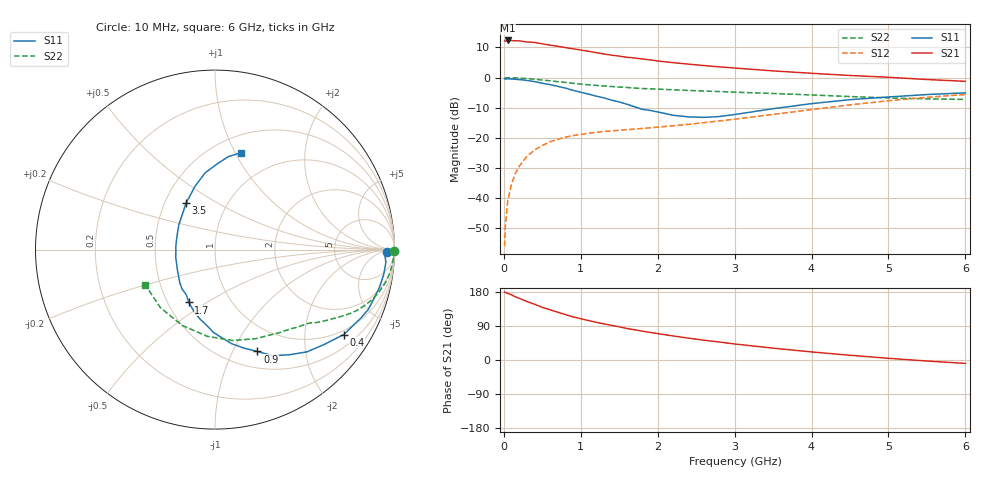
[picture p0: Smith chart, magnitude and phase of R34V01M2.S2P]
! SIEMENS Small Signal Semiconductors
! BFR181
! Si NPN RF Bipolar Junction Transistor in SOT23
! VCE = 4 V  IC = 1.2 mA
! Common Emitter S-Parameters:  May  1996
# GHz  S  MA  R  50
!  f  S11  S21  S12  S22
! GHz  MAG  ANG  MAG  ANG  MAG  ANG  MAG  ANG
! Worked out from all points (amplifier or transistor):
!   36 points, 10 MHz to 6 GHz, reference 50 ohm
!   highest |S21| = 12.3 dB at 50 MHz (marker M1)
!   |S21| within 3 dB of that: start of sweep to 957.6 MHz
!   unconditionally stable (mu >= 1): 1.924 GHz to 3.596 GHz
!   at 250 MHz: K = 0.17, MSG = 19.8 dB, |S12| = -27.7 dB
!   at 1.4 GHz: K = 0.82, MSG = 12.6 dB, |S12| = -17.7 dB
!   at 6 GHz: K = 0.87, MSG = 2.2 dB, |S12| = -5.6 dB
!   S11 on the Smith chart (normalised r, x): 10 MHz: 41, -13; 400 MHz: 0.86, -3.12; 900 MHz: 0.69, -1.25; 1.7 GHz: 0.64, -0.42; 3.5 GHz: 0.64, +0.37; 6 GHz: 0.67, +1.06
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0.01  0.956 -0.8  4.086 179.4  0.0016 93.1  0.9993 -0.4
0.02  0.9463 -1.6  4.015 178.2  0.0035 88.1  0.9892 -0.8
0.05  0.9549 -4.3  4.135 175.9  0.0089 88.3  0.9975 -2.0
0.1  0.9502 -8.4  4.114 171.9  0.0173 86.3  0.9925 -4.0
0.15  0.9404 -12.8  4.08 166.7  0.0256 81.4  0.9872 -6.1
0.2  0.9271 -17.0  4.08 162.8  0.0337 79.2  0.9814 -7.9
0.3  0.8969 -25.3  3.909 154.4  0.0493 74.3  0.9628 -11.6
0.4  0.8593 -33.4  3.833 147.1  0.063 69.4  0.9401 -15.1
0.5  0.806 -41.0  3.64 138.9  0.0747 65.3  0.9123 -18.3
0.6  0.7656 -48.1  3.456 132.6  0.0861 61.2  0.8856 -20.9
0.7  0.7172 -54.8  3.312 126.2  0.0949 58.2  0.8588 -23.3
0.9  0.6144 -67.4  3.007 113.8  0.1093 53.2  0.8052 -27.2
1.1  0.5332 -79.8  2.736 104.2  0.1193 49.7  0.7608 -30.4
1.2  0.4935 -85.4  2.596 99.5  0.1235 48.5  0.7432 -31.9
1.4  0.4229 -96.5  2.355 91.3  0.1305 46.9  0.7121 -34.4
1.7  0.3283 -116.3  2.114 79.7  0.14 46.9  0.671 -37.5
2.2  0.2375 -152.0  1.773 63.5  0.1588 48.5  0.6286 -43.5
2.6  0.2192 173.3  1.588 52.3  0.1792 50.7  0.5988 -48.7
3.5  0.3052 121.9  1.293 31.3  0.2451 52.3  0.5456 -65.5
4.5  0.4311 97.3  1.085 12.5  0.353 46.7  0.485 -95.1
5.5  0.5241 81.7  0.93 -2.7  0.4713 34.5  0.4443 -133.1
6  0.5589 75.0  0.868 -9.0  0.5248 26.7  0.4354 -153.4
